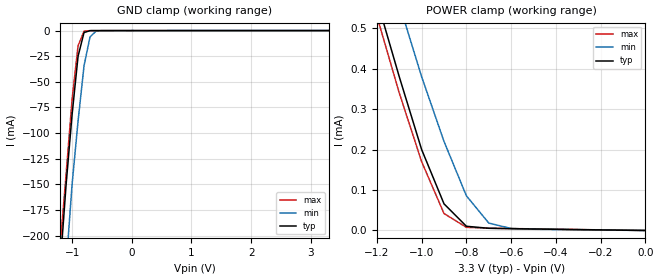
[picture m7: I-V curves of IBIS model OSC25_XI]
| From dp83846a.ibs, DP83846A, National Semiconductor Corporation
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|   Model OSC25_XI
[Model]   OSC25_XI
Model_type   Input
Polarity   Non-Inverting
Enable   Active-High
Vinl =   0.80V
Vinh =   2.00V
Vmeas =   1.50V
Cref =  10.00pF
Rref = 100.00k
C_comp   5.00pF   5.00pF   5.00pF
[Temperature Range]   25.00   0.14k   0.000
[Voltage Range]   3.30V   3.00V   3.60V
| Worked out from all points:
|   GND clamp passes 1 mA (typ) near -0.75 V on its own axis
|   POWER clamp passes 1 mA (typ) near -1.42 V on its own axis
[GND_clamp]
| voltage   I(typ)   I(min)   I(max)
-3.3V     -1.97A     -2.03A     -1.96A
-1.2V     -230mA     -300mA     -210mA
-1.1V     -150mA     -230mA     -140mA
-1V       -81.96mA   -150mA     -67.08mA
-900mV    -25.1mA    -88.33mA   -14.92mA
-800mV    -1.93mA    -34.43mA   -620uA
-700mV    -82.69uA   -6.23mA    -39.35uA
-600mV    -24uA      -590uA     -25.92uA
3.3V      7.12pA     1.71uA     -2.08uA
[POWER_clamp]
| voltage   I(typ)   I(min)   I(max)
-3.3V     4.86mA     5.01mA     4.83mA
-1.2V     570uA      750uA      530uA
-1.1V     380uA      560uA      340uA
-1V       200uA      380uA      170uA
-900mV    65.83uA    220uA      41.88uA
-800mV    10.38uA    85.67uA    7.76uA
-700mV    5.42uA     18.36uA    5.61uA
-600mV    4.5uA      4.85uA     4.76uA
0V        7.12pA     140pA      7.77pA
